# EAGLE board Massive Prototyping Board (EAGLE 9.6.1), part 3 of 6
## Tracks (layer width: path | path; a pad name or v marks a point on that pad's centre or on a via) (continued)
N$746  (via drill 0.94) (continued)
  Bottom 2.032: v140.97,119.38 v143.51,119.38 v146.05,119.38 v148.59,119.38 v151.13,119.38
N$747  (via drill 0.94)
  Bottom 2.032: v140.97,121.92 v143.51,121.92 v146.05,121.92 v148.59,121.92 v151.13,121.92
N$748  (via drill 0.94)
  Bottom 2.032: v140.97,124.46 v143.51,124.46 v146.05,124.46 v148.59,124.46 v151.13,124.46
N$749  (via drill 0.94)
  Bottom 2.032: v140.97,127 v143.51,127 v146.05,127 v148.59,127 v151.13,127
N$750  (via drill 0.94)
  Bottom 2.032: v140.97,129.54 v143.51,129.54 v146.05,129.54 v148.59,129.54 v151.13,129.54
N$751  (via drill 0.94)
  Bottom 2.032: v140.97,132.08 v143.51,132.08 v146.05,132.08 v148.59,132.08 v151.13,132.08
N$752  (via drill 0.94)
  Bottom 2.032: v140.97,134.62 v143.51,134.62 v146.05,134.62 v148.59,134.62 v151.13,134.62
N$753  (via drill 0.94)
  Bottom 2.032: v140.97,137.16 v143.51,137.16 v146.05,137.16 v148.59,137.16 v151.13,137.16
N$754  (via drill 0.94)
  Bottom 2.032: v140.97,139.7 v143.51,139.7 v146.05,139.7 v148.59,139.7 v151.13,139.7
N$755  (via drill 0.94)
  Bottom 2.032: v140.97,142.24 v143.51,142.24 v146.05,142.24 v148.59,142.24 v151.13,142.24
N$756  (via drill 0.94)
  Bottom 2.032: v140.97,144.78 v143.51,144.78 v146.05,144.78 v148.59,144.78 v151.13,144.78
N$757  (via drill 0.94)
  Bottom 2.032: v140.97,147.32 v143.51,147.32 v146.05,147.32 v148.59,147.32 v151.13,147.32
N$758  (via drill 0.94)
  Bottom 2.032: v140.97,149.86 v143.51,149.86 v146.05,149.86 v148.59,149.86 v151.13,149.86
N$759  (via drill 0.94)
  Bottom 2.032: v140.97,152.4 v143.51,152.4 v146.05,152.4 v148.59,152.4 v151.13,152.4
N$760  (via drill 0.94)
  Bottom 2.032: v140.97,154.94 v143.51,154.94 v146.05,154.94 v148.59,154.94 v151.13,154.94
N$761  (via drill 0.94)
  Bottom 2.032: v140.97,157.48 v143.51,157.48 v146.05,157.48 v148.59,157.48 v151.13,157.48
N$762  (via drill 0.94)
  Bottom 2.032: v140.97,160.02 v143.51,160.02 v146.05,160.02 v148.59,160.02 v151.13,160.02
N$763  (via drill 0.94)
  Bottom 2.032: v140.97,162.56 v143.51,162.56 v146.05,162.56 v148.59,162.56 v151.13,162.56
N$764  (via drill 0.94)
  Bottom 2.032: v140.97,165.1 v143.51,165.1 v146.05,165.1 v148.59,165.1 v151.13,165.1
N$765  (via drill 0.94)
  Bottom 2.032: v140.97,167.64 v143.51,167.64 v146.05,167.64 v148.59,167.64 v151.13,167.64
N$766  (via drill 0.94)
  Bottom 2.032: v140.97,170.18 v143.51,170.18 v146.05,170.18 v148.59,170.18 v151.13,170.18
N$767  (via drill 0.94)
  Bottom 2.032: v140.97,172.72 v143.51,172.72 v146.05,172.72 v148.59,172.72 v151.13,172.72
N$768  (via drill 0.94)
  Bottom 2.032: v140.97,175.26 v143.51,175.26 v146.05,175.26 v148.59,175.26 v151.13,175.26
N$769  (via drill 0.94)
  Bottom 2.032: v140.97,177.8 v143.51,177.8 v146.05,177.8 v148.59,177.8 v151.13,177.8
N$770  (via drill 0.94)
  Bottom 2.032: v140.97,180.34 v143.51,180.34 v146.05,180.34 v148.59,180.34 v151.13,180.34
N$771  (via drill 0.94)
  Bottom 2.032: v140.97,182.88 v143.51,182.88 v146.05,182.88 v148.59,182.88 v151.13,182.88
N$772  (via drill 0.94)
  Bottom 2.032: v140.97,185.42 v143.51,185.42 v146.05,185.42 v148.59,185.42 v151.13,185.42
N$773  (via drill 0.94)
  Bottom 2.032: v140.97,187.96 v143.51,187.96 v146.05,187.96 v148.59,187.96 v151.13,187.96
N$774  (via drill 0.94)
  Bottom 2.032: v140.97,190.5 v143.51,190.5 v146.05,190.5 v148.59,190.5 v151.13,190.5
N$775  (via drill 0.94)
  Bottom 2.032: v140.97,193.04 v143.51,193.04 v146.05,193.04 v148.59,193.04 v151.13,193.04
N$776  (via drill 0.94)
  Bottom 2.032: v140.97,195.58 v143.51,195.58 v146.05,195.58 v148.59,195.58 v151.13,195.58
N$777  (via drill 0.94)
  Bottom 2.032: v140.97,198.12 v143.51,198.12 v146.05,198.12 v148.59,198.12 v151.13,198.12
N$778  (via drill 0.94)
  Bottom 2.032: v140.97,200.66 v143.51,200.66 v146.05,200.66 v148.59,200.66 v151.13,200.66
N$779  (via drill 0.94)
  Bottom 2.032: v140.97,203.2 v143.51,203.2 v146.05,203.2 v148.59,203.2 v151.13,203.2
N$780  (via drill 0.94)
  Bottom 2.032: v140.97,205.74 v143.51,205.74 v146.05,205.74 v148.59,205.74 v151.13,205.74
N$781  (via drill 0.94)
  Bottom 2.032: v140.97,208.28 v143.51,208.28 v146.05,208.28 v148.59,208.28 v151.13,208.28
N$782  (via drill 0.94)
  Bottom 2.032: v140.97,210.82 v143.51,210.82 v146.05,210.82 v148.59,210.82 v151.13,210.82
N$783  (via drill 0.94)
  Bottom 2.032: v140.97,213.36 v143.51,213.36 v146.05,213.36 v148.59,213.36 v151.13,213.36
N$784  (via drill 0.94)
  Bottom 2.032: v140.97,215.9 v143.51,215.9 v146.05,215.9 v148.59,215.9 v151.13,215.9
N$785  (via drill 0.94)
  Bottom 2.032: v140.97,218.44 v143.51,218.44 v146.05,218.44 v148.59,218.44 v151.13,218.44
N$786  (via drill 0.94)
  Bottom 2.032: v140.97,220.98 v143.51,220.98 v146.05,220.98 v148.59,220.98 v151.13,220.98
N$787  (via drill 0.94)
  Bottom 2.032: v140.97,223.52 v143.51,223.52 v146.05,223.52 v148.59,223.52 v151.13,223.52
N$788  (via drill 0.94)
  Bottom 2.032: v140.97,226.06 v143.51,226.06 v146.05,226.06 v148.59,226.06 v151.13,226.06
N$789  (via drill 0.94)
  Bottom 2.032: v140.97,228.6 v143.51,228.6 v146.05,228.6 v148.59,228.6 v151.13,228.6
N$790  (via drill 0.94)
  Bottom 2.032: v140.97,231.14 v143.51,231.14 v146.05,231.14 v148.59,231.14 v151.13,231.14
N$791  (via drill 0.94)
  Bottom 2.032: v140.97,233.68 v143.51,233.68 v146.05,233.68 v148.59,233.68 v151.13,233.68
N$792  (via drill 0.94)
  Bottom 2.032: v140.97,236.22 v143.51,236.22 v146.05,236.22 v148.59,236.22 v151.13,236.22
N$793  (via drill 0.94)
  Bottom 2.032: v140.97,238.76 v143.51,238.76 v146.05,238.76 v148.59,238.76 v151.13,238.76
N$794  (via drill 0.94)
  Bottom 2.032: v140.97,241.3 v143.51,241.3 v146.05,241.3 v148.59,241.3 v151.13,241.3
N$795  (via drill 0.94)
  Bottom 2.032: v140.97,243.84 v143.51,243.84 v146.05,243.84 v148.59,243.84 v151.13,243.84
N$796  (via drill 0.94)
  Bottom 2.032: v140.97,246.38 v143.51,246.38 v146.05,246.38 v148.59,246.38 v151.13,246.38
N$797  (via drill 0.94)
  Bottom 2.032: v140.97,248.92 v143.51,248.92 v146.05,248.92 v148.59,248.92 v151.13,248.92
N$798  (via drill 0.94)
  Bottom 2.032: v140.97,251.46 v143.51,251.46 v146.05,251.46 v148.59,251.46 v151.13,251.46
N$799  (via drill 0.94)
  Bottom 2.032: v140.97,254 v143.51,254 v146.05,254 v148.59,254 v151.13,254
N$800  (via drill 0.94)
  Bottom 2.032: v140.97,256.54 v143.51,256.54 v146.05,256.54 v148.59,256.54 v151.13,256.54
N$801  (via drill 0.94)
  Bottom 2.032: v140.97,259.08 v143.51,259.08 v146.05,259.08 v148.59,259.08 v151.13,259.08
N$802  (via drill 0.94)
  Bottom 2.032: v140.97,261.62 v143.51,261.62 v146.05,261.62 v148.59,261.62 v151.13,261.62
N$803  (via drill 0.94)
  Bottom 2.032: v140.97,264.16 v143.51,264.16 v146.05,264.16 v148.59,264.16 v151.13,264.16
N$804  (via drill 0.94)
  Bottom 2.032: v140.97,266.7 v143.51,266.7 v146.05,266.7 v148.59,266.7 v151.13,266.7
N$805  (via drill 0.94)
  Bottom 2.032: v140.97,269.24 v143.51,269.24 v146.05,269.24 v148.59,269.24 v151.13,269.24
N$806  (via drill 0.94)
  Bottom 2.032: v140.97,271.78 v143.51,271.78 v146.05,271.78 v148.59,271.78 v151.13,271.78
N$807  (via drill 0.94)
  Bottom 2.032: v140.97,274.32 v143.51,274.32 v146.05,274.32 v148.59,274.32 v151.13,274.32
N$808  (via drill 0.94)
  Bottom 2.032: v140.97,276.86 v143.51,276.86 v146.05,276.86 v148.59,276.86 v151.13,276.86
N$809  (via drill 0.94)
  Bottom 2.032: v158.75,12.7 v161.29,12.7 v163.83,12.7 v166.37,12.7 v168.91,12.7
N$810  (via drill 0.94)
  Bottom 2.032: v158.75,15.24 v161.29,15.24 v163.83,15.24 v166.37,15.24 v168.91,15.24
N$811  (via drill 0.94)
  Bottom 2.032: v158.75,17.78 v161.29,17.78 v163.83,17.78 v166.37,17.78 v168.91,17.78
N$812  (via drill 0.94)
  Bottom 2.032: v158.75,20.32 v161.29,20.32 v163.83,20.32 v166.37,20.32 v168.91,20.32
N$813  (via drill 0.94)
  Bottom 2.032: v158.75,22.86 v161.29,22.86 v163.83,22.86 v166.37,22.86 v168.91,22.86
N$814  (via drill 0.94)
  Bottom 2.032: v158.75,25.4 v161.29,25.4 v163.83,25.4 v166.37,25.4 v168.91,25.4
N$815  (via drill 0.94)
  Bottom 2.032: v158.75,27.94 v161.29,27.94 v163.83,27.94 v166.37,27.94 v168.91,27.94
N$816  (via drill 0.94)
  Bottom 2.032: v158.75,30.48 v161.29,30.48 v163.83,30.48 v166.37,30.48 v168.91,30.48
N$817  (via drill 0.94)
  Bottom 2.032: v158.75,33.02 v161.29,33.02 v163.83,33.02 v166.37,33.02 v168.91,33.02
N$818  (via drill 0.94)
  Bottom 2.032: v158.75,35.56 v161.29,35.56 v163.83,35.56 v166.37,35.56 v168.91,35.56
N$819  (via drill 0.94)
  Bottom 2.032: v158.75,38.1 v161.29,38.1 v163.83,38.1 v166.37,38.1 v168.91,38.1
N$820  (via drill 0.94)
  Bottom 2.032: v158.75,40.64 v161.29,40.64 v163.83,40.64 v166.37,40.64 v168.91,40.64
N$821  (via drill 0.94)
  Bottom 2.032: v158.75,43.18 v161.29,43.18 v163.83,43.18 v166.37,43.18 v168.91,43.18
N$822  (via drill 0.94)
  Bottom 2.032: v158.75,45.72 v161.29,45.72 v163.83,45.72 v166.37,45.72 v168.91,45.72
N$823  (via drill 0.94)
  Bottom 2.032: v158.75,48.26 v161.29,48.26 v163.83,48.26 v166.37,48.26 v168.91,48.26
N$824  (via drill 0.94)
  Bottom 2.032: v158.75,50.8 v161.29,50.8 v163.83,50.8 v166.37,50.8 v168.91,50.8
N$825  (via drill 0.94)
  Bottom 2.032: v158.75,53.34 v161.29,53.34 v163.83,53.34 v166.37,53.34 v168.91,53.34
N$826  (via drill 0.94)
  Bottom 2.032: v158.75,55.88 v161.29,55.88 v163.83,55.88 v166.37,55.88 v168.91,55.88
N$827  (via drill 0.94)
  Bottom 2.032: v158.75,58.42 v161.29,58.42 v163.83,58.42 v166.37,58.42 v168.91,58.42
N$828  (via drill 0.94)
  Bottom 2.032: v158.75,60.96 v161.29,60.96 v163.83,60.96 v166.37,60.96 v168.91,60.96
N$829  (via drill 0.94)
  Bottom 2.032: v158.75,63.5 v161.29,63.5 v163.83,63.5 v166.37,63.5 v168.91,63.5
N$830  (via drill 0.94)
  Bottom 2.032: v158.75,66.04 v161.29,66.04 v163.83,66.04 v166.37,66.04 v168.91,66.04
N$831  (via drill 0.94)
  Bottom 2.032: v158.75,68.58 v161.29,68.58 v163.83,68.58 v166.37,68.58 v168.91,68.58
N$832  (via drill 0.94)
  Bottom 2.032: v158.75,71.12 v161.29,71.12 v163.83,71.12 v166.37,71.12 v168.91,71.12
N$833  (via drill 0.94)
  Bottom 2.032: v158.75,73.66 v161.29,73.66 v163.83,73.66 v166.37,73.66 v168.91,73.66
N$834  (via drill 0.94)
  Bottom 2.032: v158.75,76.2 v161.29,76.2 v163.83,76.2 v166.37,76.2 v168.91,76.2
N$835  (via drill 0.94)
  Bottom 2.032: v158.75,78.74 v161.29,78.74 v163.83,78.74 v166.37,78.74 v168.91,78.74
N$836  (via drill 0.94)
  Bottom 2.032: v158.75,81.28 v161.29,81.28 v163.83,81.28 v166.37,81.28 v168.91,81.28
N$837  (via drill 0.94)
  Bottom 2.032: v158.75,83.82 v161.29,83.82 v163.83,83.82 v166.37,83.82 v168.91,83.82
N$838  (via drill 0.94)
  Bottom 2.032: v158.75,86.36 v161.29,86.36 v163.83,86.36 v166.37,86.36 v168.91,86.36
N$839  (via drill 0.94)
  Bottom 2.032: v158.75,88.9 v161.29,88.9 v163.83,88.9 v166.37,88.9 v168.91,88.9
N$840  (via drill 0.94)
  Bottom 2.032: v158.75,91.44 v161.29,91.44 v163.83,91.44 v166.37,91.44 v168.91,91.44
N$841  (via drill 0.94)
  Bottom 2.032: v158.75,93.98 v161.29,93.98 v163.83,93.98 v166.37,93.98 v168.91,93.98
N$842  (via drill 0.94)
  Bottom 2.032: v158.75,96.52 v161.29,96.52 v163.83,96.52 v166.37,96.52 v168.91,96.52
N$843  (via drill 0.94)
  Bottom 2.032: v158.75,99.06 v161.29,99.06 v163.83,99.06 v166.37,99.06 v168.91,99.06
N$844  (via drill 0.94)
  Bottom 2.032: v158.75,101.6 v161.29,101.6 v163.83,101.6 v166.37,101.6 v168.91,101.6
N$845  (via drill 0.94)
  Bottom 2.032: v158.75,104.14 v161.29,104.14 v163.83,104.14 v166.37,104.14 v168.91,104.14
N$846  (via drill 0.94)
  Bottom 2.032: v158.75,106.68 v161.29,106.68 v163.83,106.68 v166.37,106.68 v168.91,106.68
N$847  (via drill 0.94)
  Bottom 2.032: v158.75,109.22 v161.29,109.22 v163.83,109.22 v166.37,109.22 v168.91,109.22
N$848  (via drill 0.94)
  Bottom 2.032: v158.75,111.76 v161.29,111.76 v163.83,111.76 v166.37,111.76 v168.91,111.76
N$849  (via drill 0.94)
  Bottom 2.032: v158.75,114.3 v161.29,114.3 v163.83,114.3 v166.37,114.3 v168.91,114.3
N$850  (via drill 0.94)
  Bottom 2.032: v158.75,116.84 v161.29,116.84 v163.83,116.84 v166.37,116.84 v168.91,116.84
N$851  (via drill 0.94)
  Bottom 2.032: v158.75,119.38 v161.29,119.38 v163.83,119.38 v166.37,119.38 v168.91,119.38
N$852  (via drill 0.94)
  Bottom 2.032: v158.75,121.92 v161.29,121.92 v163.83,121.92 v166.37,121.92 v168.91,121.92
N$853  (via drill 0.94)
  Bottom 2.032: v158.75,124.46 v161.29,124.46 v163.83,124.46 v166.37,124.46 v168.91,124.46
N$854  (via drill 0.94)
  Bottom 2.032: v158.75,127 v161.29,127 v163.83,127 v166.37,127 v168.91,127
N$855  (via drill 0.94)
  Bottom 2.032: v158.75,129.54 v161.29,129.54 v163.83,129.54 v166.37,129.54 v168.91,129.54
N$856  (via drill 0.94)
  Bottom 2.032: v158.75,132.08 v161.29,132.08 v163.83,132.08 v166.37,132.08 v168.91,132.08
N$857  (via drill 0.94)
  Bottom 2.032: v158.75,134.62 v161.29,134.62 v163.83,134.62 v166.37,134.62 v168.91,134.62
N$858  (via drill 0.94)
  Bottom 2.032: v158.75,137.16 v161.29,137.16 v163.83,137.16 v166.37,137.16 v168.91,137.16
N$859  (via drill 0.94)
  Bottom 2.032: v158.75,139.7 v161.29,139.7 v163.83,139.7 v166.37,139.7 v168.91,139.7
N$860  (via drill 0.94)
  Bottom 2.032: v158.75,142.24 v161.29,142.24 v163.83,142.24 v166.37,142.24 v168.91,142.24
N$861  (via drill 0.94)
  Bottom 2.032: v158.75,144.78 v161.29,144.78 v163.83,144.78 v166.37,144.78 v168.91,144.78
N$862  (via drill 0.94)
  Bottom 2.032: v158.75,147.32 v161.29,147.32 v163.83,147.32 v166.37,147.32 v168.91,147.32
N$863  (via drill 0.94)
  Bottom 2.032: v158.75,149.86 v161.29,149.86 v163.83,149.86 v166.37,149.86 v168.91,149.86
N$864  (via drill 0.94)
  Bottom 2.032: v158.75,152.4 v161.29,152.4 v163.83,152.4 v166.37,152.4 v168.91,152.4
N$865  (via drill 0.94)
  Bottom 2.032: v158.75,154.94 v161.29,154.94 v163.83,154.94 v166.37,154.94 v168.91,154.94
N$866  (via drill 0.94)
  Bottom 2.032: v158.75,157.48 v161.29,157.48 v163.83,157.48 v166.37,157.48 v168.91,157.48
N$867  (via drill 0.94)
  Bottom 2.032: v158.75,160.02 v161.29,160.02 v163.83,160.02 v166.37,160.02 v168.91,160.02
N$868  (via drill 0.94)
  Bottom 2.032: v158.75,162.56 v161.29,162.56 v163.83,162.56 v166.37,162.56 v168.91,162.56
N$869  (via drill 0.94)
  Bottom 2.032: v158.75,165.1 v161.29,165.1 v163.83,165.1 v166.37,165.1 v168.91,165.1
N$870  (via drill 0.94)
  Bottom 2.032: v158.75,167.64 v161.29,167.64 v163.83,167.64 v166.37,167.64 v168.91,167.64
N$871  (via drill 0.94)
  Bottom 2.032: v158.75,170.18 v161.29,170.18 v163.83,170.18 v166.37,170.18 v168.91,170.18
N$872  (via drill 0.94)
  Bottom 2.032: v158.75,172.72 v161.29,172.72 v163.83,172.72 v166.37,172.72 v168.91,172.72
N$873  (via drill 0.94)
  Bottom 2.032: v158.75,175.26 v161.29,175.26 v163.83,175.26 v166.37,175.26 v168.91,175.26
N$874  (via drill 0.94)
  Bottom 2.032: v158.75,177.8 v161.29,177.8 v163.83,177.8 v166.37,177.8 v168.91,177.8
N$875  (via drill 0.94)
  Bottom 2.032: v158.75,180.34 v161.29,180.34 v163.83,180.34 v166.37,180.34 v168.91,180.34
N$876  (via drill 0.94)
  Bottom 2.032: v158.75,182.88 v161.29,182.88 v163.83,182.88 v166.37,182.88 v168.91,182.88
N$877  (via drill 0.94)
  Bottom 2.032: v158.75,185.42 v161.29,185.42 v163.83,185.42 v166.37,185.42 v168.91,185.42
N$878  (via drill 0.94)
  Bottom 2.032: v158.75,187.96 v161.29,187.96 v163.83,187.96 v166.37,187.96 v168.91,187.96
N$879  (via drill 0.94)
  Bottom 2.032: v158.75,190.5 v161.29,190.5 v163.83,190.5 v166.37,190.5 v168.91,190.5
N$880  (via drill 0.94)
  Bottom 2.032: v158.75,193.04 v161.29,193.04 v163.83,193.04 v166.37,193.04 v168.91,193.04
N$881  (via drill 0.94)
  Bottom 2.032: v158.75,195.58 v161.29,195.58 v163.83,195.58 v166.37,195.58 v168.91,195.58
N$882  (via drill 0.94)
  Bottom 2.032: v158.75,198.12 v161.29,198.12 v163.83,198.12 v166.37,198.12 v168.91,198.12
N$883  (via drill 0.94)
  Bottom 2.032: v158.75,200.66 v161.29,200.66 v163.83,200.66 v166.37,200.66 v168.91,200.66
N$884  (via drill 0.94)
  Bottom 2.032: v158.75,203.2 v161.29,203.2 v163.83,203.2 v166.37,203.2 v168.91,203.2
N$885  (via drill 0.94)
  Bottom 2.032: v158.75,205.74 v161.29,205.74 v163.83,205.74 v166.37,205.74 v168.91,205.74
N$886  (via drill 0.94)
  Bottom 2.032: v158.75,208.28 v161.29,208.28 v163.83,208.28 v166.37,208.28 v168.91,208.28
N$887  (via drill 0.94)
  Bottom 2.032: v158.75,210.82 v161.29,210.82 v163.83,210.82 v166.37,210.82 v168.91,210.82
N$888  (via drill 0.94)
  Bottom 2.032: v158.75,213.36 v161.29,213.36 v163.83,213.36 v166.37,213.36 v168.91,213.36
N$889  (via drill 0.94)
  Bottom 2.032: v158.75,215.9 v161.29,215.9 v163.83,215.9 v166.37,215.9 v168.91,215.9
N$890  (via drill 0.94)
  Bottom 2.032: v158.75,218.44 v161.29,218.44 v163.83,218.44 v166.37,218.44 v168.91,218.44
N$891  (via drill 0.94)
  Bottom 2.032: v158.75,220.98 v161.29,220.98 v163.83,220.98 v166.37,220.98 v168.91,220.98
N$892  (via drill 0.94)
  Bottom 2.032: v158.75,223.52 v161.29,223.52 v163.83,223.52 v166.37,223.52 v168.91,223.52
N$893  (via drill 0.94)
  Bottom 2.032: v158.75,226.06 v161.29,226.06 v163.83,226.06 v166.37,226.06 v168.91,226.06
N$894  (via drill 0.94)
  Bottom 2.032: v158.75,228.6 v161.29,228.6 v163.83,228.6 v166.37,228.6 v168.91,228.6
N$895  (via drill 0.94)
  Bottom 2.032: v158.75,231.14 v161.29,231.14 v163.83,231.14 v166.37,231.14 v168.91,231.14
N$896  (via drill 0.94)
  Bottom 2.032: v158.75,233.68 v161.29,233.68 v163.83,233.68 v166.37,233.68 v168.91,233.68
N$897  (via drill 0.94)
  Bottom 2.032: v158.75,236.22 v161.29,236.22 v163.83,236.22 v166.37,236.22 v168.91,236.22
N$898  (via drill 0.94)
  Bottom 2.032: v158.75,238.76 v161.29,238.76 v163.83,238.76 v166.37,238.76 v168.91,238.76
N$899  (via drill 0.94)
  Bottom 2.032: v158.75,241.3 v161.29,241.3 v163.83,241.3 v166.37,241.3 v168.91,241.3
N$900  (via drill 0.94)
  Bottom 2.032: v158.75,243.84 v161.29,243.84 v163.83,243.84 v166.37,243.84 v168.91,243.84
N$901  (via drill 0.94)
  Bottom 2.032: v158.75,246.38 v161.29,246.38 v163.83,246.38 v166.37,246.38 v168.91,246.38
N$902  (via drill 0.94)
  Bottom 2.032: v158.75,248.92 v161.29,248.92 v163.83,248.92 v166.37,248.92 v168.91,248.92
N$903  (via drill 0.94)
  Bottom 2.032: v158.75,251.46 v161.29,251.46 v163.83,251.46 v166.37,251.46 v168.91,251.46
N$904  (via drill 0.94)
  Bottom 2.032: v158.75,254 v161.29,254 v163.83,254 v166.37,254 v168.91,254
N$905  (via drill 0.94)
  Bottom 2.032: v158.75,256.54 v161.29,256.54 v163.83,256.54 v166.37,256.54 v168.91,256.54
N$906  (via drill 0.94)
  Bottom 2.032: v158.75,259.08 v161.29,259.08 v163.83,259.08 v166.37,259.08 v168.91,259.08
N$907  (via drill 0.94)
  Bottom 2.032: v158.75,261.62 v161.29,261.62 v163.83,261.62 v166.37,261.62 v168.91,261.62
N$908  (via drill 0.94)
  Bottom 2.032: v158.75,264.16 v161.29,264.16 v163.83,264.16 v166.37,264.16 v168.91,264.16
N$909  (via drill 0.94)
  Bottom 2.032: v158.75,266.7 v161.29,266.7 v163.83,266.7 v166.37,266.7 v168.91,266.7
N$910  (via drill 0.94)
  Bottom 2.032: v158.75,269.24 v161.29,269.24 v163.83,269.24 v166.37,269.24 v168.91,269.24
N$911  (via drill 0.94)
  Bottom 2.032: v158.75,271.78 v161.29,271.78 v163.83,271.78 v166.37,271.78 v168.91,271.78
N$912  (via drill 0.94)
  Bottom 2.032: v158.75,274.32 v161.29,274.32 v163.83,274.32 v166.37,274.32 v168.91,274.32
N$913  (via drill 0.94)
  Bottom 2.032: v158.75,276.86 v161.29,276.86 v163.83,276.86 v166.37,276.86 v168.91,276.86
N$914  (via drill 0.94)
  Bottom 2.032: v171.45,12.7 v173.99,12.7 v176.53,12.7 v179.07,12.7 v181.61,12.7
N$915  (via drill 0.94)
  Bottom 2.032: v171.45,15.24 v173.99,15.24 v176.53,15.24 v179.07,15.24 v181.61,15.24
N$916  (via drill 0.94)
  Bottom 2.032: v171.45,17.78 v173.99,17.78 v176.53,17.78 v179.07,17.78 v181.61,17.78
N$917  (via drill 0.94)
  Bottom 2.032: v171.45,20.32 v173.99,20.32 v176.53,20.32 v179.07,20.32 v181.61,20.32
N$918  (via drill 0.94)
  Bottom 2.032: v171.45,22.86 v173.99,22.86 v176.53,22.86 v179.07,22.86 v181.61,22.86
N$919  (via drill 0.94)
  Bottom 2.032: v171.45,25.4 v173.99,25.4 v176.53,25.4 v179.07,25.4 v181.61,25.4
N$920  (via drill 0.94)
  Bottom 2.032: v171.45,27.94 v173.99,27.94 v176.53,27.94 v179.07,27.94 v181.61,27.94
N$921  (via drill 0.94)
  Bottom 2.032: v171.45,30.48 v173.99,30.48 v176.53,30.48 v179.07,30.48 v181.61,30.48
N$922  (via drill 0.94)
  Bottom 2.032: v171.45,33.02 v173.99,33.02 v176.53,33.02 v179.07,33.02 v181.61,33.02
N$923  (via drill 0.94)
  Bottom 2.032: v171.45,35.56 v173.99,35.56 v176.53,35.56 v179.07,35.56 v181.61,35.56
N$924  (via drill 0.94)
  Bottom 2.032: v171.45,38.1 v173.99,38.1 v176.53,38.1 v179.07,38.1 v181.61,38.1
N$925  (via drill 0.94)
  Bottom 2.032: v171.45,40.64 v173.99,40.64 v176.53,40.64 v179.07,40.64 v181.61,40.64
N$926  (via drill 0.94)
  Bottom 2.032: v171.45,43.18 v173.99,43.18 v176.53,43.18 v179.07,43.18 v181.61,43.18
N$927  (via drill 0.94)
  Bottom 2.032: v171.45,45.72 v173.99,45.72 v176.53,45.72 v179.07,45.72 v181.61,45.72
N$928  (via drill 0.94)
  Bottom 2.032: v171.45,48.26 v173.99,48.26 v176.53,48.26 v179.07,48.26 v181.61,48.26
N$929  (via drill 0.94)
  Bottom 2.032: v171.45,50.8 v173.99,50.8 v176.53,50.8 v179.07,50.8 v181.61,50.8
N$930  (via drill 0.94)
  Bottom 2.032: v171.45,53.34 v173.99,53.34 v176.53,53.34 v179.07,53.34 v181.61,53.34
N$931  (via drill 0.94)
  Bottom 2.032: v171.45,55.88 v173.99,55.88 v176.53,55.88 v179.07,55.88 v181.61,55.88
N$932  (via drill 0.94)
  Bottom 2.032: v171.45,58.42 v173.99,58.42 v176.53,58.42 v179.07,58.42 v181.61,58.42
N$933  (via drill 0.94)
  Bottom 2.032: v171.45,60.96 v173.99,60.96 v176.53,60.96 v179.07,60.96 v181.61,60.96
N$934  (via drill 0.94)
  Bottom 2.032: v171.45,63.5 v173.99,63.5 v176.53,63.5 v179.07,63.5 v181.61,63.5
N$935  (via drill 0.94)
  Bottom 2.032: v171.45,66.04 v173.99,66.04 v176.53,66.04 v179.07,66.04 v181.61,66.04
N$936  (via drill 0.94)
  Bottom 2.032: v171.45,68.58 v173.99,68.58 v176.53,68.58 v179.07,68.58 v181.61,68.58
N$937  (via drill 0.94)
  Bottom 2.032: v171.45,71.12 v173.99,71.12 v176.53,71.12 v179.07,71.12 v181.61,71.12
N$938  (via drill 0.94)
  Bottom 2.032: v171.45,73.66 v173.99,73.66 v176.53,73.66 v179.07,73.66 v181.61,73.66
N$939  (via drill 0.94)
  Bottom 2.032: v171.45,76.2 v173.99,76.2 v176.53,76.2 v179.07,76.2 v181.61,76.2
N$940  (via drill 0.94)
  Bottom 2.032: v171.45,78.74 v173.99,78.74 v176.53,78.74 v179.07,78.74 v181.61,78.74
N$941  (via drill 0.94)
  Bottom 2.032: v171.45,81.28 v173.99,81.28 v176.53,81.28 v179.07,81.28 v181.61,81.28
N$942  (via drill 0.94)
  Bottom 2.032: v171.45,83.82 v173.99,83.82 v176.53,83.82 v179.07,83.82 v181.61,83.82
N$943  (via drill 0.94)
  Bottom 2.032: v171.45,86.36 v173.99,86.36 v176.53,86.36 v179.07,86.36 v181.61,86.36
N$944  (via drill 0.94)
  Bottom 2.032: v171.45,88.9 v173.99,88.9 v176.53,88.9 v179.07,88.9 v181.61,88.9
N$945  (via drill 0.94)
  Bottom 2.032: v171.45,91.44 v173.99,91.44 v176.53,91.44 v179.07,91.44 v181.61,91.44
N$946  (via drill 0.94)
  Bottom 2.032: v171.45,93.98 v173.99,93.98 v176.53,93.98 v179.07,93.98 v181.61,93.98
N$947  (via drill 0.94)
  Bottom 2.032: v171.45,96.52 v173.99,96.52 v176.53,96.52 v179.07,96.52 v181.61,96.52
N$948  (via drill 0.94)
  Bottom 2.032: v171.45,99.06 v173.99,99.06 v176.53,99.06 v179.07,99.06 v181.61,99.06
N$949  (via drill 0.94)
  Bottom 2.032: v171.45,101.6 v173.99,101.6 v176.53,101.6 v179.07,101.6 v181.61,101.6
N$950  (via drill 0.94)
  Bottom 2.032: v171.45,104.14 v173.99,104.14 v176.53,104.14 v179.07,104.14 v181.61,104.14
N$951  (via drill 0.94)
  Bottom 2.032: v171.45,106.68 v173.99,106.68 v176.53,106.68 v179.07,106.68 v181.61,106.68
N$952  (via drill 0.94)
  Bottom 2.032: v171.45,109.22 v173.99,109.22 v176.53,109.22 v179.07,109.22 v181.61,109.22
N$953  (via drill 0.94)
  Bottom 2.032: v171.45,111.76 v173.99,111.76 v176.53,111.76 v179.07,111.76 v181.61,111.76
N$954  (via drill 0.94)
  Bottom 2.032: v171.45,114.3 v173.99,114.3 v176.53,114.3 v179.07,114.3 v181.61,114.3
N$955  (via drill 0.94)
  Bottom 2.032: v171.45,116.84 v173.99,116.84 v176.53,116.84 v179.07,116.84 v181.61,116.84
N$956  (via drill 0.94)
  Bottom 2.032: v171.45,119.38 v173.99,119.38 v176.53,119.38 v179.07,119.38 v181.61,119.38
N$957  (via drill 0.94)
  Bottom 2.032: v171.45,121.92 v173.99,121.92 v176.53,121.92 v179.07,121.92 v181.61,121.92
N$958  (via drill 0.94)
  Bottom 2.032: v171.45,124.46 v173.99,124.46 v176.53,124.46 v179.07,124.46 v181.61,124.46
N$959  (via drill 0.94)
  Bottom 2.032: v171.45,127 v173.99,127 v176.53,127 v179.07,127 v181.61,127
N$960  (via drill 0.94)
  Bottom 2.032: v171.45,129.54 v173.99,129.54 v176.53,129.54 v179.07,129.54 v181.61,129.54
N$961  (via drill 0.94)
  Bottom 2.032: v171.45,132.08 v173.99,132.08 v176.53,132.08 v179.07,132.08 v181.61,132.08
N$962  (via drill 0.94)
  Bottom 2.032: v171.45,134.62 v173.99,134.62 v176.53,134.62 v179.07,134.62 v181.61,134.62
N$963  (via drill 0.94)
  Bottom 2.032: v171.45,137.16 v173.99,137.16 v176.53,137.16 v179.07,137.16 v181.61,137.16
N$964  (via drill 0.94)
  Bottom 2.032: v171.45,139.7 v173.99,139.7 v176.53,139.7 v179.07,139.7 v181.61,139.7
N$965  (via drill 0.94)
  Bottom 2.032: v171.45,142.24 v173.99,142.24 v176.53,142.24 v179.07,142.24 v181.61,142.24
N$966  (via drill 0.94)
  Bottom 2.032: v171.45,144.78 v173.99,144.78 v176.53,144.78 v179.07,144.78 v181.61,144.78
N$967  (via drill 0.94)
  Bottom 2.032: v171.45,147.32 v173.99,147.32 v176.53,147.32 v179.07,147.32 v181.61,147.32
N$968  (via drill 0.94)
  Bottom 2.032: v171.45,149.86 v173.99,149.86 v176.53,149.86 v179.07,149.86 v181.61,149.86
N$969  (via drill 0.94)
  Bottom 2.032: v171.45,152.4 v173.99,152.4 v176.53,152.4 v179.07,152.4 v181.61,152.4
N$970  (via drill 0.94)
  Bottom 2.032: v171.45,154.94 v173.99,154.94 v176.53,154.94 v179.07,154.94 v181.61,154.94
N$971  (via drill 0.94)
  Bottom 2.032: v171.45,157.48 v173.99,157.48 v176.53,157.48 v179.07,157.48 v181.61,157.48
N$972  (via drill 0.94)
  Bottom 2.032: v171.45,160.02 v173.99,160.02 v176.53,160.02 v179.07,160.02 v181.61,160.02
N$973  (via drill 0.94)
  Bottom 2.032: v171.45,162.56 v173.99,162.56 v176.53,162.56 v179.07,162.56 v181.61,162.56
N$974  (via drill 0.94)
  Bottom 2.032: v171.45,165.1 v173.99,165.1 v176.53,165.1 v179.07,165.1 v181.61,165.1
N$975  (via drill 0.94)
  Bottom 2.032: v171.45,167.64 v173.99,167.64 v176.53,167.64 v179.07,167.64 v181.61,167.64
N$976  (via drill 0.94)
  Bottom 2.032: v171.45,170.18 v173.99,170.18 v176.53,170.18 v179.07,170.18 v181.61,170.18
N$977  (via drill 0.94)
  Bottom 2.032: v171.45,172.72 v173.99,172.72 v176.53,172.72 v179.07,172.72 v181.61,172.72
N$978  (via drill 0.94)
  Bottom 2.032: v171.45,175.26 v173.99,175.26 v176.53,175.26 v179.07,175.26 v181.61,175.26
N$979  (via drill 0.94)
  Bottom 2.032: v171.45,177.8 v173.99,177.8 v176.53,177.8 v179.07,177.8 v181.61,177.8
N$980  (via drill 0.94)
  Bottom 2.032: v171.45,180.34 v173.99,180.34 v176.53,180.34 v179.07,180.34 v181.61,180.34
N$981  (via drill 0.94)
  Bottom 2.032: v171.45,182.88 v173.99,182.88 v176.53,182.88 v179.07,182.88 v181.61,182.88
N$982  (via drill 0.94)
  Bottom 2.032: v171.45,185.42 v173.99,185.42 v176.53,185.42 v179.07,185.42 v181.61,185.42
N$983  (via drill 0.94)
  Bottom 2.032: v171.45,187.96 v173.99,187.96 v176.53,187.96 v179.07,187.96 v181.61,187.96
N$984  (via drill 0.94)
  Bottom 2.032: v171.45,190.5 v173.99,190.5 v176.53,190.5 v179.07,190.5 v181.61,190.5
N$985  (via drill 0.94)
  Bottom 2.032: v171.45,193.04 v173.99,193.04 v176.53,193.04 v179.07,193.04 v181.61,193.04
N$986  (via drill 0.94)
  Bottom 2.032: v171.45,195.58 v173.99,195.58 v176.53,195.58 v179.07,195.58 v181.61,195.58
N$987  (via drill 0.94)
  Bottom 2.032: v171.45,198.12 v173.99,198.12 v176.53,198.12 v179.07,198.12 v181.61,198.12
N$988  (via drill 0.94)
  Bottom 2.032: v171.45,200.66 v173.99,200.66 v176.53,200.66 v179.07,200.66 v181.61,200.66
N$989  (via drill 0.94)
  Bottom 2.032: v171.45,203.2 v173.99,203.2 v176.53,203.2 v179.07,203.2 v181.61,203.2
N$990  (via drill 0.94)
  Bottom 2.032: v171.45,205.74 v173.99,205.74 v176.53,205.74 v179.07,205.74 v181.61,205.74
N$991  (via drill 0.94)
  Bottom 2.032: v171.45,208.28 v173.99,208.28 v176.53,208.28 v179.07,208.28 v181.61,208.28
N$992  (via drill 0.94)
  Bottom 2.032: v171.45,210.82 v173.99,210.82 v176.53,210.82 v179.07,210.82 v181.61,210.82
N$993  (via drill 0.94)
  Bottom 2.032: v171.45,213.36 v173.99,213.36 v176.53,213.36 v179.07,213.36 v181.61,213.36
N$994  (via drill 0.94)
  Bottom 2.032: v171.45,215.9 v173.99,215.9 v176.53,215.9 v179.07,215.9 v181.61,215.9
N$995  (via drill 0.94)
  Bottom 2.032: v171.45,218.44 v173.99,218.44 v176.53,218.44 v179.07,218.44 v181.61,218.44
N$996  (via drill 0.94)
  Bottom 2.032: v171.45,220.98 v173.99,220.98 v176.53,220.98 v179.07,220.98 v181.61,220.98
N$997  (via drill 0.94)
  Bottom 2.032: v171.45,223.52 v173.99,223.52 v176.53,223.52 v179.07,223.52 v181.61,223.52
N$998  (via drill 0.94)
  Bottom 2.032: v171.45,226.06 v173.99,226.06 v176.53,226.06 v179.07,226.06 v181.61,226.06
N$999  (via drill 0.94)
  Bottom 2.032: v171.45,228.6 v173.99,228.6 v176.53,228.6 v179.07,228.6 v181.61,228.6
N$1000  (via drill 0.94)
  Bottom 2.032: v171.45,231.14 v173.99,231.14 v176.53,231.14 v179.07,231.14 v181.61,231.14
N$1001  (via drill 0.94)
  Bottom 2.032: v171.45,233.68 v173.99,233.68 v176.53,233.68 v179.07,233.68 v181.61,233.68
N$1002  (via drill 0.94)
  Bottom 2.032: v171.45,236.22 v173.99,236.22 v176.53,236.22 v179.07,236.22 v181.61,236.22
N$1003  (via drill 0.94)
  Bottom 2.032: v171.45,238.76 v173.99,238.76 v176.53,238.76 v179.07,238.76 v181.61,238.76
N$1004  (via drill 0.94)
  Bottom 2.032: v171.45,241.3 v173.99,241.3 v176.53,241.3 v179.07,241.3 v181.61,241.3
N$1005  (via drill 0.94)
  Bottom 2.032: v171.45,243.84 v173.99,243.84 v176.53,243.84 v179.07,243.84 v181.61,243.84
N$1006  (via drill 0.94)
  Bottom 2.032: v171.45,246.38 v173.99,246.38 v176.53,246.38 v179.07,246.38 v181.61,246.38
N$1007  (via drill 0.94)
  Bottom 2.032: v171.45,248.92 v173.99,248.92 v176.53,248.92 v179.07,248.92 v181.61,248.92
N$1008  (via drill 0.94)
  Bottom 2.032: v171.45,251.46 v173.99,251.46 v176.53,251.46 v179.07,251.46 v181.61,251.46
N$1009  (via drill 0.94)
  Bottom 2.032: v171.45,254 v173.99,254 v176.53,254 v179.07,254 v181.61,254
N$1010  (via drill 0.94)
  Bottom 2.032: v171.45,256.54 v173.99,256.54 v176.53,256.54 v179.07,256.54 v181.61,256.54
N$1011  (via drill 0.94)
  Bottom 2.032: v171.45,259.08 v173.99,259.08 v176.53,259.08 v179.07,259.08 v181.61,259.08
N$1012  (via drill 0.94)
  Bottom 2.032: v171.45,261.62 v173.99,261.62 v176.53,261.62 v179.07,261.62 v181.61,261.62
N$1013  (via drill 0.94)
  Bottom 2.032: v171.45,264.16 v173.99,264.16 v176.53,264.16 v179.07,264.16 v181.61,264.16
N$1014  (via drill 0.94)
  Bottom 2.032: v171.45,266.7 v173.99,266.7 v176.53,266.7 v179.07,266.7 v181.61,266.7
N$1015  (via drill 0.94)
  Bottom 2.032: v171.45,269.24 v173.99,269.24 v176.53,269.24 v179.07,269.24 v181.61,269.24
N$1016  (via drill 0.94)
  Bottom 2.032: v171.45,271.78 v173.99,271.78 v176.53,271.78 v179.07,271.78 v181.61,271.78
N$1017  (via drill 0.94)
  Bottom 2.032: v171.45,274.32 v173.99,274.32 v176.53,274.32 v179.07,274.32 v181.61,274.32
N$1018  (via drill 0.94)
  Bottom 2.032: v171.45,276.86 v173.99,276.86 v176.53,276.86 v179.07,276.86 v181.61,276.86
N$1019  (via drill 0.94)
  Bottom 2.032: v189.23,12.7 v191.77,12.7 v194.31,12.7 v196.85,12.7 v199.39,12.7
N$1020  (via drill 0.94)
  Bottom 2.032: v189.23,15.24 v191.77,15.24 v194.31,15.24 v196.85,15.24 v199.39,15.24
N$1021  (via drill 0.94)
  Bottom 2.032: v189.23,17.78 v191.77,17.78 v194.31,17.78 v196.85,17.78 v199.39,17.78
N$1022  (via drill 0.94)
  Bottom 2.032: v189.23,20.32 v191.77,20.32 v194.31,20.32 v196.85,20.32 v199.39,20.32
N$1023  (via drill 0.94)
  Bottom 2.032: v189.23,22.86 v191.77,22.86 v194.31,22.86 v196.85,22.86 v199.39,22.86
N$1024  (via drill 0.94)
  Bottom 2.032: v189.23,25.4 v191.77,25.4 v194.31,25.4 v196.85,25.4 v199.39,25.4
N$1025  (via drill 0.94)
  Bottom 2.032: v189.23,27.94 v191.77,27.94 v194.31,27.94 v196.85,27.94 v199.39,27.94
N$1026  (via drill 0.94)
  Bottom 2.032: v189.23,30.48 v191.77,30.48 v194.31,30.48 v196.85,30.48 v199.39,30.48
N$1027  (via drill 0.94)
  Bottom 2.032: v189.23,33.02 v191.77,33.02 v194.31,33.02 v196.85,33.02 v199.39,33.02
N$1028  (via drill 0.94)
  Bottom 2.032: v189.23,35.56 v191.77,35.56 v194.31,35.56 v196.85,35.56 v199.39,35.56
N$1029  (via drill 0.94)
  Bottom 2.032: v189.23,38.1 v191.77,38.1 v194.31,38.1 v196.85,38.1 v199.39,38.1
N$1030  (via drill 0.94)
  Bottom 2.032: v189.23,40.64 v191.77,40.64 v194.31,40.64 v196.85,40.64 v199.39,40.64
N$1031  (via drill 0.94)
  Bottom 2.032: v189.23,43.18 v191.77,43.18 v194.31,43.18 v196.85,43.18 v199.39,43.18
N$1032  (via drill 0.94)
  Bottom 2.032: v189.23,45.72 v191.77,45.72 v194.31,45.72 v196.85,45.72 v199.39,45.72
N$1033  (via drill 0.94)
  Bottom 2.032: v189.23,48.26 v191.77,48.26 v194.31,48.26 v196.85,48.26 v199.39,48.26
N$1034  (via drill 0.94)
  Bottom 2.032: v189.23,50.8 v191.77,50.8 v194.31,50.8 v196.85,50.8 v199.39,50.8
N$1035  (via drill 0.94)
  Bottom 2.032: v189.23,53.34 v191.77,53.34 v194.31,53.34 v196.85,53.34 v199.39,53.34
N$1036  (via drill 0.94)
  Bottom 2.032: v189.23,55.88 v191.77,55.88 v194.31,55.88 v196.85,55.88 v199.39,55.88
N$1037  (via drill 0.94)
  Bottom 2.032: v189.23,58.42 v191.77,58.42 v194.31,58.42 v196.85,58.42 v199.39,58.42
N$1038  (via drill 0.94)
  Bottom 2.032: v189.23,60.96 v191.77,60.96 v194.31,60.96 v196.85,60.96 v199.39,60.96
N$1039  (via drill 0.94)
  Bottom 2.032: v189.23,63.5 v191.77,63.5 v194.31,63.5 v196.85,63.5 v199.39,63.5
N$1040  (via drill 0.94)
  Bottom 2.032: v189.23,66.04 v191.77,66.04 v194.31,66.04 v196.85,66.04 v199.39,66.04
N$1041  (via drill 0.94)
  Bottom 2.032: v189.23,68.58 v191.77,68.58 v194.31,68.58 v196.85,68.58 v199.39,68.58
N$1042  (via drill 0.94)
  Bottom 2.032: v189.23,71.12 v191.77,71.12 v194.31,71.12 v196.85,71.12 v199.39,71.12
N$1043  (via drill 0.94)
  Bottom 2.032: v189.23,73.66 v191.77,73.66 v194.31,73.66 v196.85,73.66 v199.39,73.66
N$1044  (via drill 0.94)
  Bottom 2.032: v189.23,76.2 v191.77,76.2 v194.31,76.2 v196.85,76.2 v199.39,76.2
N$1045  (via drill 0.94)
  Bottom 2.032: v189.23,78.74 v191.77,78.74 v194.31,78.74 v196.85,78.74 v199.39,78.74
N$1046  (via drill 0.94)
  Bottom 2.032: v189.23,81.28 v191.77,81.28 v194.31,81.28 v196.85,81.28 v199.39,81.28
N$1047  (via drill 0.94)
  Bottom 2.032: v189.23,83.82 v191.77,83.82 v194.31,83.82 v196.85,83.82 v199.39,83.82
N$1048  (via drill 0.94)
  Bottom 2.032: v189.23,86.36 v191.77,86.36 v194.31,86.36 v196.85,86.36 v199.39,86.36
N$1049  (via drill 0.94)
  Bottom 2.032: v189.23,88.9 v191.77,88.9 v194.31,88.9 v196.85,88.9 v199.39,88.9
N$1050  (via drill 0.94)
  Bottom 2.032: v189.23,91.44 v191.77,91.44 v194.31,91.44 v196.85,91.44 v199.39,91.44
N$1051  (via drill 0.94)
  Bottom 2.032: v189.23,93.98 v191.77,93.98 v194.31,93.98 v196.85,93.98 v199.39,93.98
N$1052  (via drill 0.94)
  Bottom 2.032: v189.23,96.52 v191.77,96.52 v194.31,96.52 v196.85,96.52 v199.39,96.52
N$1053  (via drill 0.94)
  Bottom 2.032: v189.23,99.06 v191.77,99.06 v194.31,99.06 v196.85,99.06 v199.39,99.06
N$1054  (via drill 0.94)
  Bottom 2.032: v189.23,101.6 v191.77,101.6 v194.31,101.6 v196.85,101.6 v199.39,101.6
N$1055  (via drill 0.94)
  Bottom 2.032: v189.23,104.14 v191.77,104.14 v194.31,104.14 v196.85,104.14 v199.39,104.14
N$1056  (via drill 0.94)
  Bottom 2.032: v189.23,106.68 v191.77,106.68 v194.31,106.68 v196.85,106.68 v199.39,106.68
N$1057  (via drill 0.94)
  Bottom 2.032: v189.23,109.22 v191.77,109.22 v194.31,109.22 v196.85,109.22 v199.39,109.22
N$1058  (via drill 0.94)
  Bottom 2.032: v189.23,111.76 v191.77,111.76 v194.31,111.76 v196.85,111.76 v199.39,111.76
N$1059  (via drill 0.94)
  Bottom 2.032: v189.23,114.3 v191.77,114.3 v194.31,114.3 v196.85,114.3 v199.39,114.3
N$1060  (via drill 0.94)
  Bottom 2.032: v189.23,116.84 v191.77,116.84 v194.31,116.84 v196.85,116.84 v199.39,116.84
N$1061  (via drill 0.94)
  Bottom 2.032: v189.23,119.38 v191.77,119.38 v194.31,119.38 v196.85,119.38 v199.39,119.38
N$1062  (via drill 0.94)
  Bottom 2.032: v189.23,121.92 v191.77,121.92 v194.31,121.92 v196.85,121.92 v199.39,121.92
N$1063  (via drill 0.94)
  Bottom 2.032: v189.23,124.46 v191.77,124.46 v194.31,124.46 v196.85,124.46 v199.39,124.46
N$1064  (via drill 0.94)
  Bottom 2.032: v189.23,127 v191.77,127 v194.31,127 v196.85,127 v199.39,127
N$1065  (via drill 0.94)
  Bottom 2.032: v189.23,129.54 v191.77,129.54 v194.31,129.54 v196.85,129.54 v199.39,129.54
N$1066  (via drill 0.94)
  Bottom 2.032: v189.23,132.08 v191.77,132.08 v194.31,132.08 v196.85,132.08 v199.39,132.08
N$1067  (via drill 0.94)
  Bottom 2.032: v189.23,134.62 v191.77,134.62 v194.31,134.62 v196.85,134.62 v199.39,134.62
N$1068  (via drill 0.94)
  Bottom 2.032: v189.23,137.16 v191.77,137.16 v194.31,137.16 v196.85,137.16 v199.39,137.16
N$1069  (via drill 0.94)
  Bottom 2.032: v189.23,139.7 v191.77,139.7 v194.31,139.7 v196.85,139.7 v199.39,139.7
N$1070  (via drill 0.94)
  Bottom 2.032: v189.23,142.24 v191.77,142.24 v194.31,142.24 v196.85,142.24 v199.39,142.24
N$1071  (via drill 0.94)
  Bottom 2.032: v189.23,144.78 v191.77,144.78 v194.31,144.78 v196.85,144.78 v199.39,144.78
N$1072  (via drill 0.94)
  Bottom 2.032: v189.23,147.32 v191.77,147.32 v194.31,147.32 v196.85,147.32 v199.39,147.32
N$1073  (via drill 0.94)
  Bottom 2.032: v189.23,149.86 v191.77,149.86 v194.31,149.86 v196.85,149.86 v199.39,149.86
N$1074  (via drill 0.94)
  Bottom 2.032: v189.23,152.4 v191.77,152.4 v194.31,152.4 v196.85,152.4 v199.39,152.4
N$1075  (via drill 0.94)
  Bottom 2.032: v189.23,154.94 v191.77,154.94 v194.31,154.94 v196.85,154.94 v199.39,154.94
N$1076  (via drill 0.94)
  Bottom 2.032: v189.23,157.48 v191.77,157.48 v194.31,157.48 v196.85,157.48 v199.39,157.48
N$1077  (via drill 0.94)
  Bottom 2.032: v189.23,160.02 v191.77,160.02 v194.31,160.02 v196.85,160.02 v199.39,160.02
N$1078  (via drill 0.94)
  Bottom 2.032: v189.23,162.56 v191.77,162.56 v194.31,162.56 v196.85,162.56 v199.39,162.56
N$1079  (via drill 0.94)
  Bottom 2.032: v189.23,165.1 v191.77,165.1 v194.31,165.1 v196.85,165.1 v199.39,165.1
N$1080  (via drill 0.94)
  Bottom 2.032: v189.23,167.64 v191.77,167.64 v194.31,167.64 v196.85,167.64 v199.39,167.64
N$1081  (via drill 0.94)
  Bottom 2.032: v189.23,170.18 v191.77,170.18 v194.31,170.18 v196.85,170.18 v199.39,170.18
N$1082  (via drill 0.94)
  Bottom 2.032: v189.23,172.72 v191.77,172.72 v194.31,172.72 v196.85,172.72 v199.39,172.72
N$1083  (via drill 0.94)
  Bottom 2.032: v189.23,175.26 v191.77,175.26 v194.31,175.26 v196.85,175.26 v199.39,175.26
N$1084  (via drill 0.94)
  Bottom 2.032: v189.23,177.8 v191.77,177.8 v194.31,177.8 v196.85,177.8 v199.39,177.8
N$1085  (via drill 0.94)
  Bottom 2.032: v189.23,180.34 v191.77,180.34 v194.31,180.34 v196.85,180.34 v199.39,180.34
N$1086  (via drill 0.94)
  Bottom 2.032: v189.23,182.88 v191.77,182.88 v194.31,182.88 v196.85,182.88 v199.39,182.88
N$1087  (via drill 0.94)
  Bottom 2.032: v189.23,185.42 v191.77,185.42 v194.31,185.42 v196.85,185.42 v199.39,185.42
N$1088  (via drill 0.94)
  Bottom 2.032: v189.23,187.96 v191.77,187.96 v194.31,187.96 v196.85,187.96 v199.39,187.96
N$1089  (via drill 0.94)
  Bottom 2.032: v189.23,190.5 v191.77,190.5 v194.31,190.5 v196.85,190.5 v199.39,190.5
N$1090  (via drill 0.94)
  Bottom 2.032: v189.23,193.04 v191.77,193.04 v194.31,193.04 v196.85,193.04 v199.39,193.04
N$1091  (via drill 0.94)
  Bottom 2.032: v189.23,195.58 v191.77,195.58 v194.31,195.58 v196.85,195.58 v199.39,195.58
N$1092  (via drill 0.94)
  Bottom 2.032: v189.23,198.12 v191.77,198.12 v194.31,198.12 v196.85,198.12 v199.39,198.12
N$1093  (via drill 0.94)
  Bottom 2.032: v189.23,200.66 v191.77,200.66 v194.31,200.66 v196.85,200.66 v199.39,200.66
N$1094  (via drill 0.94)
  Bottom 2.032: v189.23,203.2 v191.77,203.2 v194.31,203.2 v196.85,203.2 v199.39,203.2
N$1095  (via drill 0.94)
  Bottom 2.032: v189.23,205.74 v191.77,205.74 v194.31,205.74 v196.85,205.74 v199.39,205.74
N$1096  (via drill 0.94)
  Bottom 2.032: v189.23,208.28 v191.77,208.28 v194.31,208.28 v196.85,208.28 v199.39,208.28
N$1097  (via drill 0.94)
  Bottom 2.032: v189.23,210.82 v191.77,210.82 v194.31,210.82 v196.85,210.82 v199.39,210.82
N$1098  (via drill 0.94)
  Bottom 2.032: v189.23,213.36 v191.77,213.36 v194.31,213.36 v196.85,213.36 v199.39,213.36
N$1099  (via drill 0.94)
  Bottom 2.032: v189.23,215.9 v191.77,215.9 v194.31,215.9 v196.85,215.9 v199.39,215.9
N$1100  (via drill 0.94)
  Bottom 2.032: v189.23,218.44 v191.77,218.44 v194.31,218.44 v196.85,218.44 v199.39,218.44
N$1101  (via drill 0.94)
  Bottom 2.032: v189.23,220.98 v191.77,220.98 v194.31,220.98 v196.85,220.98 v199.39,220.98
N$1102  (via drill 0.94)
  Bottom 2.032: v189.23,223.52 v191.77,223.52 v194.31,223.52 v196.85,223.52 v199.39,223.52
N$1103  (via drill 0.94)
  Bottom 2.032: v189.23,226.06 v191.77,226.06 v194.31,226.06 v196.85,226.06 v199.39,226.06
N$1104  (via drill 0.94)
  Bottom 2.032: v189.23,228.6 v191.77,228.6 v194.31,228.6 v196.85,228.6 v199.39,228.6
N$1105  (via drill 0.94)
  Bottom 2.032: v189.23,231.14 v191.77,231.14 v194.31,231.14 v196.85,231.14 v199.39,231.14
N$1106  (via drill 0.94)
  Bottom 2.032: v189.23,233.68 v191.77,233.68 v194.31,233.68 v196.85,233.68 v199.39,233.68
N$1107  (via drill 0.94)
  Bottom 2.032: v189.23,236.22 v191.77,236.22 v194.31,236.22 v196.85,236.22 v199.39,236.22
N$1108  (via drill 0.94)
  Bottom 2.032: v189.23,238.76 v191.77,238.76 v194.31,238.76 v196.85,238.76 v199.39,238.76
N$1109  (via drill 0.94)
  Bottom 2.032: v189.23,241.3 v191.77,241.3 v194.31,241.3 v196.85,241.3 v199.39,241.3
N$1110  (via drill 0.94)
  Bottom 2.032: v189.23,243.84 v191.77,243.84 v194.31,243.84 v196.85,243.84 v199.39,243.84
N$1111  (via drill 0.94)
  Bottom 2.032: v189.23,246.38 v191.77,246.38 v194.31,246.38 v196.85,246.38 v199.39,246.38
N$1112  (via drill 0.94)
  Bottom 2.032: v189.23,248.92 v191.77,248.92 v194.31,248.92 v196.85,248.92 v199.39,248.92
N$1113  (via drill 0.94)
  Bottom 2.032: v189.23,251.46 v191.77,251.46 v194.31,251.46 v196.85,251.46 v199.39,251.46
N$1114  (via drill 0.94)
  Bottom 2.032: v189.23,254 v191.77,254 v194.31,254 v196.85,254 v199.39,254
N$1115  (via drill 0.94)
  Bottom 2.032: v189.23,256.54 v191.77,256.54 v194.31,256.54 v196.85,256.54 v199.39,256.54
N$1116  (via drill 0.94)
  Bottom 2.032: v189.23,259.08 v191.77,259.08 v194.31,259.08 v196.85,259.08 v199.39,259.08
N$1117  (via drill 0.94)
  Bottom 2.032: v189.23,261.62 v191.77,261.62 v194.31,261.62 v196.85,261.62 v199.39,261.62
N$1118  (via drill 0.94)
  Bottom 2.032: v189.23,264.16 v191.77,264.16 v194.31,264.16 v196.85,264.16 v199.39,264.16
N$1119  (via drill 0.94)
  Bottom 2.032: v189.23,266.7 v191.77,266.7 v194.31,266.7 v196.85,266.7 v199.39,266.7
N$1120  (via drill 0.94)
  Bottom 2.032: v189.23,269.24 v191.77,269.24 v194.31,269.24 v196.85,269.24 v199.39,269.24
N$1121  (via drill 0.94)
  Bottom 2.032: v189.23,271.78 v191.77,271.78 v194.31,271.78 v196.85,271.78 v199.39,271.78
N$1122  (via drill 0.94)
  Bottom 2.032: v189.23,274.32 v191.77,274.32 v194.31,274.32 v196.85,274.32 v199.39,274.32
N$1123  (via drill 0.94)
  Bottom 2.032: v189.23,276.86 v191.77,276.86 v194.31,276.86 v196.85,276.86 v199.39,276.86
N$1124  (via drill 0.94)
  Bottom 2.032: v201.93,12.7 v204.47,12.7 v207.01,12.7 v209.55,12.7 v212.09,12.7
N$1125  (via drill 0.94)
  Bottom 2.032: v201.93,15.24 v204.47,15.24 v207.01,15.24 v209.55,15.24 v212.09,15.24
N$1126  (via drill 0.94)
  Bottom 2.032: v201.93,17.78 v204.47,17.78 v207.01,17.78 v209.55,17.78 v212.09,17.78
N$1127  (via drill 0.94)
  Bottom 2.032: v201.93,20.32 v204.47,20.32 v207.01,20.32 v209.55,20.32 v212.09,20.32
N$1128  (via drill 0.94)
  Bottom 2.032: v201.93,22.86 v204.47,22.86 v207.01,22.86 v209.55,22.86 v212.09,22.86
N$1129  (via drill 0.94)
  Bottom 2.032: v201.93,25.4 v204.47,25.4 v207.01,25.4 v209.55,25.4 v212.09,25.4
N$1130  (via drill 0.94)
  Bottom 2.032: v201.93,27.94 v204.47,27.94 v207.01,27.94 v209.55,27.94 v212.09,27.94
N$1131  (via drill 0.94)
  Bottom 2.032: v201.93,30.48 v204.47,30.48 v207.01,30.48 v209.55,30.48 v212.09,30.48
N$1132  (via drill 0.94)
  Bottom 2.032: v201.93,33.02 v204.47,33.02 v207.01,33.02 v209.55,33.02 v212.09,33.02
N$1133  (via drill 0.94)
  Bottom 2.032: v201.93,35.56 v204.47,35.56 v207.01,35.56 v209.55,35.56 v212.09,35.56
N$1134  (via drill 0.94)
  Bottom 2.032: v201.93,38.1 v204.47,38.1 v207.01,38.1 v209.55,38.1 v212.09,38.1
N$1135  (via drill 0.94)
  Bottom 2.032: v201.93,40.64 v204.47,40.64 v207.01,40.64 v209.55,40.64 v212.09,40.64
N$1136  (via drill 0.94)
  Bottom 2.032: v201.93,43.18 v204.47,43.18 v207.01,43.18 v209.55,43.18 v212.09,43.18
N$1137  (via drill 0.94)
  Bottom 2.032: v201.93,45.72 v204.47,45.72 v207.01,45.72 v209.55,45.72 v212.09,45.72
N$1138  (via drill 0.94)
  Bottom 2.032: v201.93,48.26 v204.47,48.26 v207.01,48.26 v209.55,48.26 v212.09,48.26
N$1139  (via drill 0.94)
  Bottom 2.032: v201.93,50.8 v204.47,50.8 v207.01,50.8 v209.55,50.8 v212.09,50.8
N$1140  (via drill 0.94)
  Bottom 2.032: v201.93,53.34 v204.47,53.34 v207.01,53.34 v209.55,53.34 v212.09,53.34
N$1141  (via drill 0.94)
  Bottom 2.032: v201.93,55.88 v204.47,55.88 v207.01,55.88 v209.55,55.88 v212.09,55.88
N$1142  (via drill 0.94)
  Bottom 2.032: v201.93,58.42 v204.47,58.42 v207.01,58.42 v209.55,58.42 v212.09,58.42
N$1143  (via drill 0.94)
  Bottom 2.032: v201.93,60.96 v204.47,60.96 v207.01,60.96 v209.55,60.96 v212.09,60.96
N$1144  (via drill 0.94)
  Bottom 2.032: v201.93,63.5 v204.47,63.5 v207.01,63.5 v209.55,63.5 v212.09,63.5
N$1145  (via drill 0.94)
  Bottom 2.032: v201.93,66.04 v204.47,66.04 v207.01,66.04 v209.55,66.04 v212.09,66.04
N$1146  (via drill 0.94)
  Bottom 2.032: v201.93,68.58 v204.47,68.58 v207.01,68.58 v209.55,68.58 v212.09,68.58
N$1147  (via drill 0.94)
  Bottom 2.032: v201.93,71.12 v204.47,71.12 v207.01,71.12 v209.55,71.12 v212.09,71.12
N$1148  (via drill 0.94)
  Bottom 2.032: v201.93,73.66 v204.47,73.66 v207.01,73.66 v209.55,73.66 v212.09,73.66
N$1149  (via drill 0.94)
  Bottom 2.032: v201.93,76.2 v204.47,76.2 v207.01,76.2 v209.55,76.2 v212.09,76.2
N$1150  (via drill 0.94)
  Bottom 2.032: v201.93,78.74 v204.47,78.74 v207.01,78.74 v209.55,78.74 v212.09,78.74
N$1151  (via drill 0.94)
  Bottom 2.032: v201.93,81.28 v204.47,81.28 v207.01,81.28 v209.55,81.28 v212.09,81.28
N$1152  (via drill 0.94)
  Bottom 2.032: v201.93,83.82 v204.47,83.82 v207.01,83.82 v209.55,83.82 v212.09,83.82
N$1153  (via drill 0.94)
  Bottom 2.032: v201.93,86.36 v204.47,86.36 v207.01,86.36 v209.55,86.36 v212.09,86.36
N$1154  (via drill 0.94)
  Bottom 2.032: v201.93,88.9 v204.47,88.9 v207.01,88.9 v209.55,88.9 v212.09,88.9
N$1155  (via drill 0.94)
  Bottom 2.032: v201.93,91.44 v204.47,91.44 v207.01,91.44 v209.55,91.44 v212.09,91.44
N$1156  (via drill 0.94)
  Bottom 2.032: v201.93,93.98 v204.47,93.98 v207.01,93.98 v209.55,93.98 v212.09,93.98
N$1157  (via drill 0.94)
  Bottom 2.032: v201.93,96.52 v204.47,96.52 v207.01,96.52 v209.55,96.52 v212.09,96.52
N$1158  (via drill 0.94)
  Bottom 2.032: v201.93,99.06 v204.47,99.06 v207.01,99.06 v209.55,99.06 v212.09,99.06
N$1159  (via drill 0.94)
  Bottom 2.032: v201.93,101.6 v204.47,101.6 v207.01,101.6 v209.55,101.6 v212.09,101.6
N$1160  (via drill 0.94)
  Bottom 2.032: v201.93,104.14 v204.47,104.14 v207.01,104.14 v209.55,104.14 v212.09,104.14
N$1161  (via drill 0.94)
  Bottom 2.032: v201.93,106.68 v204.47,106.68 v207.01,106.68 v209.55,106.68 v212.09,106.68
N$1162  (via drill 0.94)
  Bottom 2.032: v201.93,109.22 v204.47,109.22 v207.01,109.22 v209.55,109.22 v212.09,109.22
N$1163  (via drill 0.94)
  Bottom 2.032: v201.93,111.76 v204.47,111.76 v207.01,111.76 v209.55,111.76 v212.09,111.76
N$1164  (via drill 0.94)
  Bottom 2.032: v201.93,114.3 v204.47,114.3 v207.01,114.3 v209.55,114.3 v212.09,114.3
N$1165  (via drill 0.94)
  Bottom 2.032: v201.93,116.84 v204.47,116.84 v207.01,116.84 v209.55,116.84 v212.09,116.84
N$1166  (via drill 0.94)
  Bottom 2.032: v201.93,119.38 v204.47,119.38 v207.01,119.38 v209.55,119.38 v212.09,119.38
N$1167  (via drill 0.94)
  Bottom 2.032: v201.93,121.92 v204.47,121.92 v207.01,121.92 v209.55,121.92 v212.09,121.92
N$1168  (via drill 0.94)
  Bottom 2.032: v201.93,124.46 v204.47,124.46 v207.01,124.46 v209.55,124.46 v212.09,124.46
N$1169  (via drill 0.94)
  Bottom 2.032: v201.93,127 v204.47,127 v207.01,127 v209.55,127 v212.09,127
N$1170  (via drill 0.94)
  Bottom 2.032: v201.93,129.54 v204.47,129.54 v207.01,129.54 v209.55,129.54 v212.09,129.54
N$1171  (via drill 0.94)
  Bottom 2.032: v201.93,132.08 v204.47,132.08 v207.01,132.08 v209.55,132.08 v212.09,132.08
N$1172  (via drill 0.94)
  Bottom 2.032: v201.93,134.62 v204.47,134.62 v207.01,134.62 v209.55,134.62 v212.09,134.62
N$1173  (via drill 0.94)
  Bottom 2.032: v201.93,137.16 v204.47,137.16 v207.01,137.16 v209.55,137.16 v212.09,137.16
N$1174  (via drill 0.94)
  Bottom 2.032: v201.93,139.7 v204.47,139.7 v207.01,139.7 v209.55,139.7 v212.09,139.7
N$1175  (via drill 0.94)
  Bottom 2.032: v201.93,142.24 v204.47,142.24 v207.01,142.24 v209.55,142.24 v212.09,142.24
N$1176  (via drill 0.94)
  Bottom 2.032: v201.93,144.78 v204.47,144.78 v207.01,144.78 v209.55,144.78 v212.09,144.78
N$1177  (via drill 0.94)
  Bottom 2.032: v201.93,147.32 v204.47,147.32 v207.01,147.32 v209.55,147.32 v212.09,147.32
N$1178  (via drill 0.94)
  Bottom 2.032: v201.93,149.86 v204.47,149.86 v207.01,149.86 v209.55,149.86 v212.09,149.86
N$1179  (via drill 0.94)
  Bottom 2.032: v201.93,152.4 v204.47,152.4 v207.01,152.4 v209.55,152.4 v212.09,152.4
N$1180  (via drill 0.94)
  Bottom 2.032: v201.93,154.94 v204.47,154.94 v207.01,154.94 v209.55,154.94 v212.09,154.94
N$1181  (via drill 0.94)
  Bottom 2.032: v201.93,157.48 v204.47,157.48 v207.01,157.48 v209.55,157.48 v212.09,157.48
N$1182  (via drill 0.94)
  Bottom 2.032: v201.93,160.02 v204.47,160.02 v207.01,160.02 v209.55,160.02 v212.09,160.02
N$1183  (via drill 0.94)
  Bottom 2.032: v201.93,162.56 v204.47,162.56 v207.01,162.56 v209.55,162.56 v212.09,162.56
N$1184  (via drill 0.94)
  Bottom 2.032: v201.93,165.1 v204.47,165.1 v207.01,165.1 v209.55,165.1 v212.09,165.1
N$1185  (via drill 0.94)
  Bottom 2.032: v201.93,167.64 v204.47,167.64 v207.01,167.64 v209.55,167.64 v212.09,167.64
N$1186  (via drill 0.94)
  Bottom 2.032: v201.93,170.18 v204.47,170.18 v207.01,170.18 v209.55,170.18 v212.09,170.18
N$1187  (via drill 0.94)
